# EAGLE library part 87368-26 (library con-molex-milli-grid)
RECEPTACAL
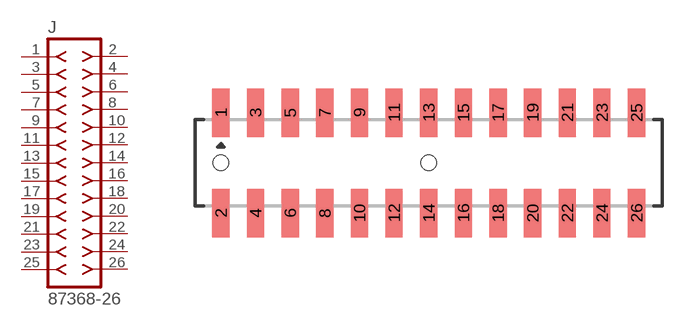
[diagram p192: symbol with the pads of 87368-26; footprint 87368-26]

Designator prefix J

## 87368-26  [87368-26]
1  1  pas
2  2  pas
3  3  pas
4  4  pas
5  5  pas
6  6  pas
7  7  pas
8  8  pas
9  9  pas
10  10  pas
11  11  pas
12  12  pas
13  13  pas
14  14  pas
15  15  pas
16  16  pas
17  17  pas
18  18  pas
19  19  pas
20  20  pas
21  21  pas
22  22  pas
23  23  pas
24  24  pas
25  25  pas
26  26  pas

## Footprint 87368-26 (pad centres in mm)
RECEPTACAL SMD Dual Row, Side Entry
smd 1 x 2.8: 1 -12,2.9; 2 -12,-2.9; 3 -10,2.9; 4 -10,-2.9; 5 -8,2.9; 6 -8,-2.9; 7 -6,2.9; 8 -6,-2.9; 9 -4,2.9; 10 -4,-2.9; 11 -2,2.9; 12 -2,-2.9; 13 0,2.9; 14 0,-2.9; 15 2,2.9; 16 2,-2.9; 17 4,2.9; 18 4,-2.9; 19 6,2.9; 20 6,-2.9; 21 8,2.9; 22 8,-2.9; 23 10,2.9; 24 10,-2.9; 25 12,2.9; 26 12,-2.9
hole 0.914 at -12,0
hole 0.914 at 0,0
